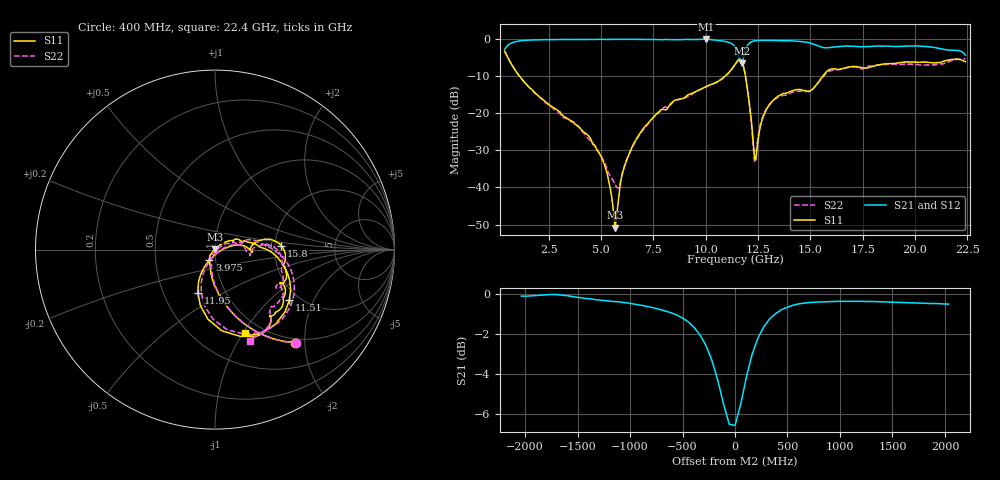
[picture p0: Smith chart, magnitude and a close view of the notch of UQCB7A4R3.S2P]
!  Part Number  UQCB7A4R3	Mounting Orientation: Vertical
!  Description: RF capacitors
!  Application: Coupling, Bypass, Tuning, DC Block
!  Filters, Matching
# GHZ S DB R 50
! Freq  |S11|  S11 Ph  |S21|  S21 Ph  |S12|  S12 Ph  |S22|  S22 Ph
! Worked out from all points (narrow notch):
!   401 points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, 400 MHz to 22.4 GHz, reference 50 ohm
!   highest |S21| = -0.01 dB at 10.03 GHz (marker M1); lowest = -6.6 dB at 11.73 GHz (marker M2)
!   notch at M2: 6.1 dB deep, 347 MHz wide at half that depth
!   lowest |S11| = -50.9 dB at 5.68 GHz (marker M3), VSWR 1.01, Z = 49.8 + j0.212 ohm
!   |S11| at or under -10 dB: 1.111 GHz to 10.92 GHz (9.813 GHz wide, 163 % of centre); 11.9 GHz to 15.59 GHz (3.687 GHz wide, 26.8 % of centre)
!   |S22| runs from -40.1 to -3.3 dB; largest |S21 - S12| = 0.0046
!   S11 on the Smith chart (normalised r, x): 400 MHz: 0.92, -1.81; 3.975 GHz: 0.93, -0.10; 11.51 GHz: 1.77, -1.33; 11.95 GHz: 0.74, -0.38; 15.8 GHz: 2.16, +0.11; 22.4 GHz: 0.83, -1.02
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0.4  -3.28 -49.2  -2.81 40.6  -2.81 40.5  -3.25 -49.1
1.335  -11.55 -83.5  -0.36 5.9  -0.37 5.9  -11.61 -83.3
3.975  -23.83 -119.5  -0.14 -23.8  -0.15 -23.8  -23.93 -119.3
4.085  -24.56 -121.0  -0.14 -24.7  -0.13 -24.7  -24.75 -120.0
5.13  -33.31 -136.4  -0.09 -33.7  -0.09 -33.7  -32.76 -109.2
5.68  -50.85 132.0  -0.10 -38.0  -0.10 -38.0  -39.34 -55.0
6.065  -35.45 49.9  -0.08 -41.3  -0.07 -41.3  -35.25 14.0
6.395  -30.34 44.9  -0.08 -44.0  -0.07 -44.0  -30.50 25.9
7.77  -19.60 28.7  -0.15 -55.3  -0.15 -55.3  -19.85 22.0
10.025  -12.77 7.3  -0.01 -75.6  0.00 -75.6  -12.82 12.8
11.4  -6.88 -23.0  -2.06 -99.2  -2.05 -99.3  -6.84 -17.9
11.51  -6.00 -34.3  -3.31 -102.0  -3.30 -102.0  -5.91 -29.5
11.73  -5.94 -73.6  -6.57 -76.2  -6.56 -76.2  -5.91 -69.3
11.95  -11.78 -111.9  -2.17 -64.5  -2.16 -64.5  -11.87 -107.5
12.28  -28.45 -104.0  -0.55 -77.0  -0.55 -77.1  -29.57 -95.8
12.39  -32.60 -35.2  -0.44 -79.9  -0.44 -79.9  -31.87 -19.4
12.72  -21.38 11.7  -0.35 -86.0  -0.35 -86.0  -20.94 15.4
13.215  -16.54 9.4  -0.39 -92.5  -0.38 -92.6  -16.64 8.4
15.085  -13.60 6.8  -1.25 -114.2  -1.24 -114.2  -13.63 0.3
15.8  -8.65 3.4  -2.36 -113.6  -2.34 -113.8  -9.04 -1.4
18.77  -6.63 -34.5  -1.93 -130.5  -1.94 -130.7  -6.79 -34.3
22.4  -6.10 -70.4  -4.35 -166.2  -4.35 -166.3  -5.26 -69.1
